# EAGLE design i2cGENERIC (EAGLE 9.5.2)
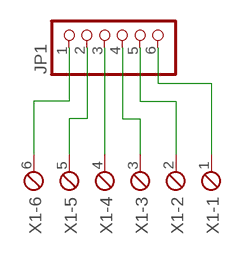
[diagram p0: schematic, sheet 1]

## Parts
JP1  PINHD-1X6  [1X06]
X1  MPT6  [6POL254]

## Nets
N$1: JP1.1 X1.6
N$2: JP1.2 X1.5
N$3: JP1.3 X1.4
N$4: JP1.4 X1.3
N$5: JP1.5 X1.2
N$6: JP1.6 X1.1

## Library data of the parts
JP1 = pinhead:PINHD-1X6: PIN HEADER
X1 = con-phoenix-254:MPT6: PHOENIX CONNECTOR; OC_FARNELL: unknown; OC_NEWARK: unknown

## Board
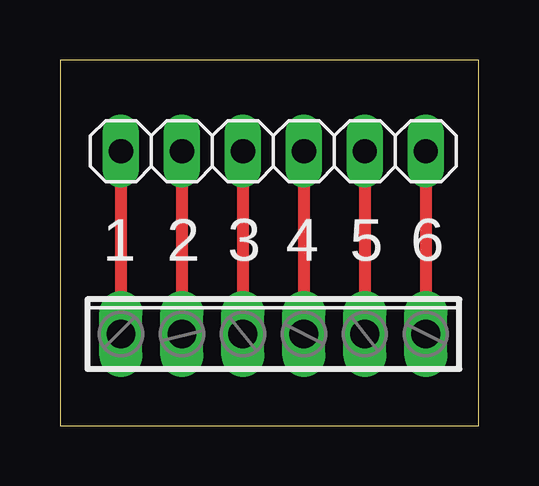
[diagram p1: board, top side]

Size 17.45 x 15.23 mm. Coordinates in mm from the lower left corner, seen from the top.
Outline: 0,0 17.45,0 17.45,15.23 0,15.23 0,0
Copper layers (1*16): Top 0.035mm / dielectric 1.5mm / Bottom 0.035mm
Design rules "default": minimum track width 6mil, minimum drill 0.35mm, track to track 6mil, track to pad 6mil, pad to pad 6mil, via to via 6mil, smd to smd 6mil, copper to edge 40mil, drill to drill 6mil, minimum pad ring 10mil, minimum via ring 8mil, stop-mask expansion 4mil, vias tented up to drill 0mil, thermal gap 10mil

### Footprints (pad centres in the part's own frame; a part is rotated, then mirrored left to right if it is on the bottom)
1X06 = drill 1.016 long: 1 -6.35,0; 2 -3.81,0; 3 -1.27,0; 4 1.27,0; 5 3.81,0; 6 6.35,0
6POL254 = drill 1.2 pad 1.778 long: 1 -6.35,0; 2 -3.81,0; 3 -1.27,0; 4 1.27,0; 5 3.81,0; 6 6.35,0

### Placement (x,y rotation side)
JP1  8.89,11.43 180 top
X1  8.89,3.81 0 top

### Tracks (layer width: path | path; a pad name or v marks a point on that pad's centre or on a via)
N$1
  Top 0.508: JP1.1 X1.6
N$2
  Top 0.508: JP1.2 X1.5
N$3
  Top 0.508: JP1.3 X1.4
N$4
  Top 0.508: JP1.4 X1.3
N$5
  Top 0.508: JP1.5 X1.2
N$6
  Top 0.508: JP1.6 X1.1

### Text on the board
tPlace: 1 | 2 | 3 | 4 | 5 | 6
